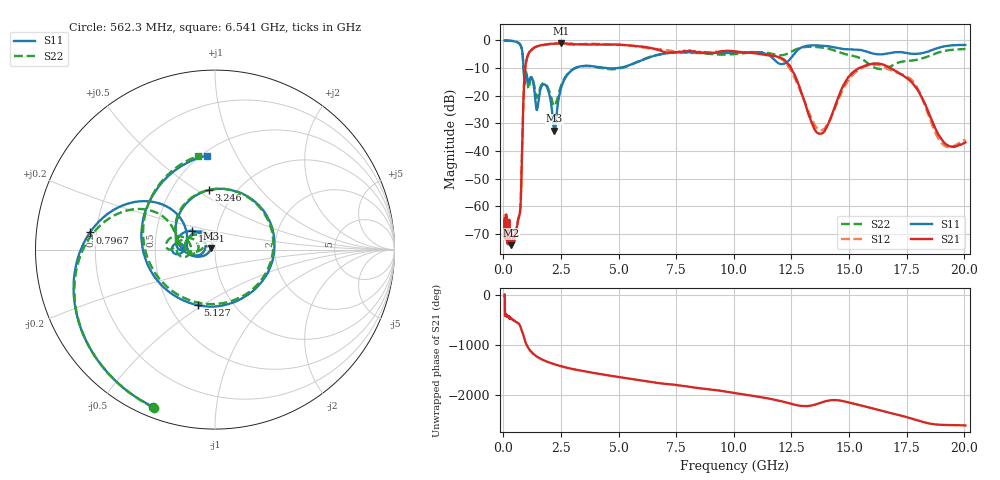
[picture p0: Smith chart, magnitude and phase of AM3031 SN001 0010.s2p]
# Hz S DB R 50
!freq MagS11 AngS11 MagS21 AngS21 MagS12 AngS12 MagS22 AngS22
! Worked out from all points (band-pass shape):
!   1601 points, 50 MHz to 20.05 GHz, reference 50 ohm
!   highest |S21| = -1.05 dB at 2.507 GHz (marker M1); lowest = -74.1 dB at 329.1 MHz (marker M2)
!   |S21| within 3 dB of the highest: 1.14 GHz to 6.925 GHz (5.785 GHz wide, 143 % of centre); 9.398 GHz to 10.16 GHz (758.9 MHz wide, 7.76 % of centre)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
!   lowest |S11| = -32.7 dB at 2.215 GHz (marker M3), VSWR 1.05, Z = 47.9 + j0.82 ohm
!   |S11| at or under -10 dB: 871.5 MHz to 3.111 GHz (2.24 GHz wide, 112 % of centre); 4.442 GHz to 4.953 GHz (510.6 MHz wide, 10.9 % of centre)
!   |S22| runs from -23.7 to 0.0 dB; largest |S21 - S12| = 0.082
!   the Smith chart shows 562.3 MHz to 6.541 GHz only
!   S11 on the Smith chart (normalised r, x): 562.3 MHz: 0.04, -0.68; 796.7 MHz: 0.18, +0.07; 1.301 GHz: 0.76, +0.16; 3.246 GHz: 0.75, +0.56; 5.127 GHz: 0.69, -0.48; 6.541 GHz: 0.53, +0.77
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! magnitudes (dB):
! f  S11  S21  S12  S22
! 50 MHz  0.0  -69.6  -67.9  0.0
! 135.9 MHz  0.0  -70.2  -69.6  0.0
! 329.1 MHz  -0.1  -74.1  -73.5  -0.1
! 369.6 MHz  -0.2  -73.1  -73.5  -0.2
! 562.3 MHz  -0.5  -68.0  -68.2  -0.5
! 725.5 MHz  -1.5  -61.7  -61.4  -1.5
! 796.7 MHz  -3.1  -44.0  -43.7  -3.2
! 894.8 MHz  -14.0  -15.6  -15.7  -12.9
! 1.005 GHz  -12.5  -7.0  -6.9  -12.4
! 1.301 GHz  -15.6  -2.8  -2.9  -15.0
! 1.879 GHz  -16.8  -1.5  -1.5  -16.3
! 2.215 GHz  -32.7  -1.1  -1.1  -23.7
! 2.507 GHz  -17.1  -1.0  -1.1  -16.3
! 2.722 GHz  -13.0  -1.1  -1.3  -12.8
! 3.246 GHz  -9.6  -1.4  -1.5  -9.6
! 5.127 GHz  -9.8  -1.6  -1.6  -10.0
! 6.541 GHz  -5.6  -3.0  -3.0  -5.5
! 7.402 GHz  -4.4  -4.3  -4.0  -4.4
! 11.91 GHz  -8.2  -6.0  -6.0  -5.3
! 13.73 GHz  -1.8  -33.8  -32.5  -2.5
! 16.44 GHz  -5.0  -8.6  -9.3  -10.4
! 20.05 GHz  -1.6  -36.9  -35.9  -3.1
